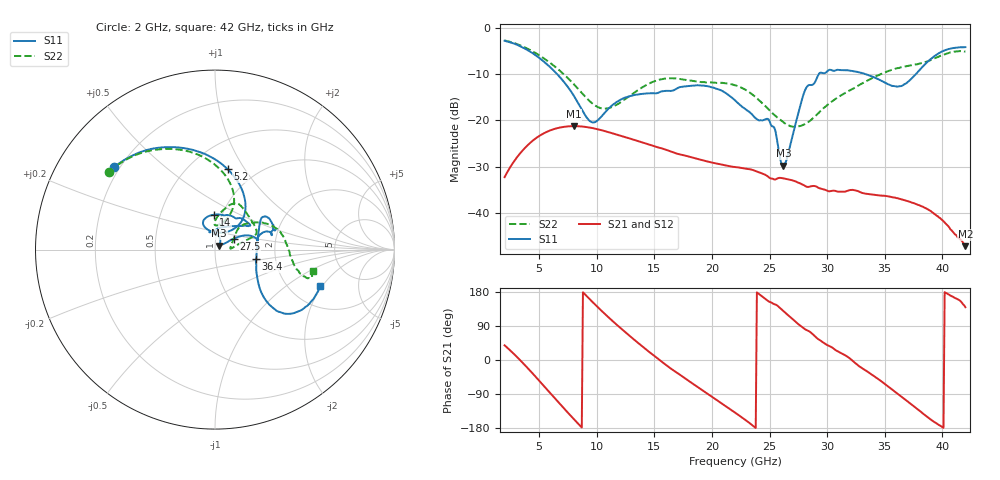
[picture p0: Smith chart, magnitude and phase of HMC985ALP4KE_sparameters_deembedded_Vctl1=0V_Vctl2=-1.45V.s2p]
!s2p File: Measurements: S11, S21, S12, S22
# GHz S dB R 50.0
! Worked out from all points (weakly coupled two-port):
!   401 points, 2 GHz to 42 GHz, reference 50 ohm
!   highest |S21| = -21.22 dB at 8 GHz (marker M1); lowest = -47.2 dB at 42 GHz (marker M2)
!   lowest |S11| = -29.8 dB at 26.2 GHz (marker M3), VSWR 1.07, Z = 52.4 + j2.3 ohm
!   |S11| at or under -10 dB: 6.568 GHz to 29.27 GHz (22.7 GHz wide, 127 % of centre); 33.35 GHz to 37.69 GHz (4.342 GHz wide, 12.2 % of centre)
!   |S22| runs from -21.4 to -2.7 dB; largest |S21 - S12| = 0.00012
!   S11 on the Smith chart (normalised r, x): 2 GHz: 0.18, +0.35; 5.2 GHz: 0.74, +0.84; 14 GHz: 0.91, +0.37; 27.5 GHz: 1.22, +0.15; 36.4 GHz: 1.58, -0.18; 42 GHz: 2.90, -1.91
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2  -2.78 140.8  -32.24 38.7  -32.24 38.7  -2.71 143.7
3.5  -4.13 113.2  -26.66 -5.2  -26.66 -5.2  -3.92 118.6
5.2  -6.86 81.2  -23.05 -61.4  -23.05 -61.4  -6.22 92.4
8  -14.62 46.2  -21.21 -155.7  -21.22 -155.7  -12.13 66.6
8.7  -17.64 52.0  -21.30 -178.1  -21.30 -178.1  -14.04 67.7
9.7  -20.43 84.6  -21.67 151.0  -21.68 151.0  -16.49 76.4
10.8  -18.02 112.2  -22.36 118.7  -22.36 118.7  -17.42 88.5
14  -14.23 92.5  -24.77 34.8  -24.77 34.8  -12.76 77.2
15.4  -13.94 73.0  -25.86 1.4  -25.86 1.4  -11.20 68.6
19.4  -12.52 34.5  -28.72 -84.7  -28.73 -84.7  -11.74 37.6
22  -15.64 52.3  -30.05 -138.6  -30.07 -138.6  -12.38 20.0
25  -20.15 98.1  -32.40 153.5  -32.42 153.5  -17.82 12.0
26.2  -29.78 42.6  -32.50 129.0  -32.51 128.9  -20.40 5.0
27.5  -18.38 29.9  -33.46 94.5  -33.44 94.6  -21.29 6.9
28.1  -13.35 20.8  -34.17 80.7  -34.18 80.7  -20.75 14.1
28.7  -12.30 12.9  -34.17 69.5  -34.15 69.6  -19.65 22.1
31  -9.07 23.3  -35.38 21.6  -35.38 21.6  -14.86 42.3
33.3  -9.95 34.4  -35.80 -26.9  -35.80 -26.8  -11.67 35.1
35.4  -12.27 12.3  -36.45 -72.4  -36.45 -72.3  -9.26 22.5
36.4  -12.57 -12.9  -37.00 -95.7  -37.02 -95.9  -8.49 15.2
39.5  -5.81 -43.3  -40.57 -167.4  -40.55 -167.5  -6.37 -14.3
42  -4.14 -19.0  -47.16 139.3  -46.98 139.7  -5.08 -12.5
